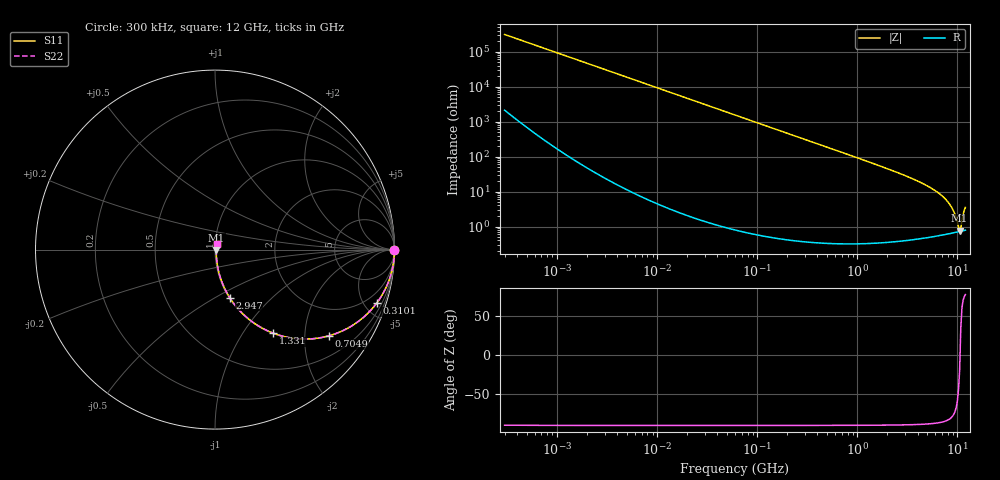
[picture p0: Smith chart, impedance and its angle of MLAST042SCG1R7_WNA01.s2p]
! MLAST042SCG1R7_WNA01  S-PARAMETER MODEL  ( General Type )
! Model Generated by TAIYO YUDEN Corporation (http://www.ty-top.com)
! Version 1.0
! TAIYO YUDEN Control No. 150820
! Copyright(c) 2015 TAIYO YUDEN CO.,LTD. All Rights Reserved.
! Product Description (link to TY-COMPAS)
! https://ds.yuden.co.jp/TYCOMPAS/or/detail?pn=MLAST042SCG1R7AWNA01&u=M
! Products Name : Multilayer Ceramic Capacitors
! Characteristics :
!  Capacitance : 1.7 pF , Rated Voltage : 25V , TCC : CG / C0G
!  Case Size : 0.4 x 0.2 / 0.016 x 0.008 [mm/inch] , Thickness : 0.2 / 0.008 [mm/inch]
!  (Conditions: Temperature = 25 degC , DC Bias Current/Voltage = 0A / 0V)
! External Node Assignments :
!  1  o---| |---o  2
! GND o---------o GND
! Frequency Range : 0.3MHz  -  12000MHz  [ 401 STEP ]
# MHz S RI R 50
! Freq[MHz].  S11 Real  S11 Imag  S21 Real  S21 Imag  S12 Real  S12 Imag  S22 Real  S22 Imag
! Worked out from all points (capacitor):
!   401 points, 300 kHz to 12 GHz, reference 50 ohm
!   read as one part in series: C = 1.71 pF near 316.3 kHz
!   lowest |Z| = 765 mohm at 10.51 GHz (marker M1)
!   series resonance near 10.61 GHz, so ESL is about 130 pH
!   S11 on the Smith chart (normalised r, x): 300 kHz: open; 310.1 MHz: 1.01, -6.00; 704.9 MHz: 1.01, -2.63; 1.331 GHz: 1.01, -1.38; 2.947 GHz: 1.01, -0.58; 12 GHz: 1.02, +0.07
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0.3  1 -0.000322  2.31e-06 0.000322  2.31e-06 0.000322  1 -0.000322
1.769972  1 -0.0019  5.72e-06 0.0019  5.72e-06 0.0019  1 -0.0019
10.44266  0.9999 -0.0112  0.000131 0.0112  0.000131 0.0112  0.9999 -0.0112
60  0.9958 -0.0641  0.00416 0.0641  0.00416 0.0641  0.9958 -0.0641
143.8206  0.9766 -0.1508  0.0234 0.1508  0.0234 0.1508  0.9766 -0.1508
310.0777  0.8998 -0.2996  0.1002 0.2996  0.1002 0.2996  0.8998 -0.2996
353.9943  0.8733 -0.332  0.1267 0.332  0.1267 0.332  0.8733 -0.332
704.9044  0.6336 -0.4806  0.3664 0.4806  0.3664 0.4806  0.6336 -0.4806
1331.232  0.3226 -0.4651  0.6774 0.4651  0.6774 0.4651  0.3226 -0.4651
2088.533  0.1575 -0.3601  0.8425 0.3601  0.8425 0.3601  0.1575 -0.3601
2947.191  0.0816 -0.2671  0.9184 0.2671  0.9184 0.2671  0.0816 -0.2671
5006.236  0.0251 -0.1407  0.9749 0.1407  0.9749 0.1407  0.0251 -0.1407
7064.448  0.011 -0.0727  0.989 0.0727  0.989 0.0727  0.011 -0.0727
7854.144  0.00889 -0.0534  0.9911 0.0534  0.9911 0.0534  0.00889 -0.0534
8732.115  0.0076 -0.0346  0.9924 0.0346  0.9924 0.0346  0.0076 -0.0346
9454.42  0.00713 -0.0207  0.9929 0.0207  0.9929 0.0207  0.00713 -0.0207
10236.47  0.00708 -0.00693  0.9929 0.00693  0.9929 0.00693  0.00708 -0.00693
10511.28  0.00716 -0.00255  0.9928 0.00255  0.9928 0.00255  0.00716 -0.00255
10793.46  0.0073 0.00484  0.9927 -0.00484  0.9927 -0.00484  0.0073 0.00484
11083.22  0.00756 0.0127  0.9924 -0.0127  0.9924 -0.0127  0.00756 0.0127
11686.27  0.00841 0.0273  0.9916 -0.0273  0.9916 -0.0273  0.00841 0.0273
12000  0.00894 0.0338  0.9911 -0.0338  0.9911 -0.0338  0.00894 0.0338
